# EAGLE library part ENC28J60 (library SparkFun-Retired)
Microchip SPI 10Base ethernet IC Prototype by abe, 2010. Dead?
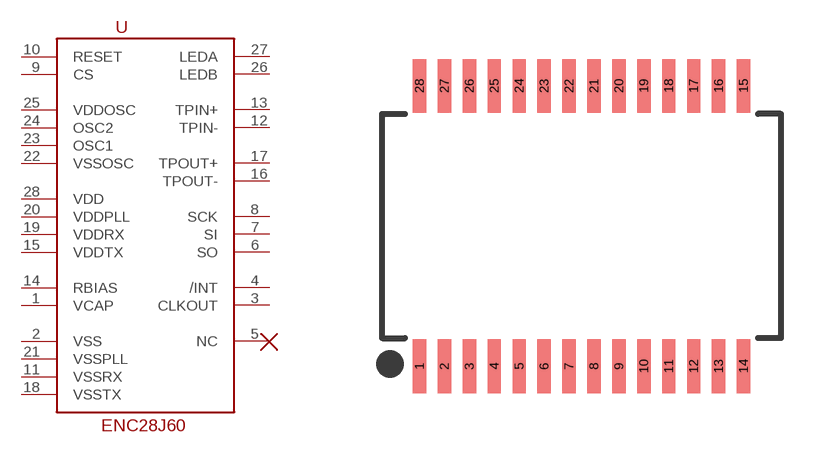
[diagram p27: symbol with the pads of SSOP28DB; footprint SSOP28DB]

Designator prefix U

## ENC28J60 (PROD_ID: IC-09541; VALUE: ENC28J60)  [SSOP28DB]
1  VCAP
2  VSS
3  CLKOUT
4  /INT
5  NC
6  SO
7  SI
8  SCK
9  CS
10  RESET
11  VSSRX
12  TPIN-
13  TPIN+
14  RBIAS
15  VDDTX
16  TPOUT-
17  TPOUT+
18  VSSTX
19  VDDRX
20  VDDPLL
21  VSSPLL
22  VSSOSC
23  OSC1
24  OSC2
25  VDDOSC
26  LEDB
27  LEDA
28  VDD

## Footprint SSOP28DB (pad centres in mm)
Small Shrink Outline Package
smd 0.348 x 1.397: 1 -4.225,-3.656; 2 -3.575,-3.656; 3 -2.925,-3.656; 4 -2.275,-3.656; 5 -1.625,-3.656; 6 -0.975,-3.656; 7 -0.325,-3.656; 8 0.325,-3.656; 9 0.975,-3.656; 10 1.625,-3.656; 11 2.275,-3.656; 12 2.925,-3.656; 13 3.575,-3.656; 14 4.225,-3.656; 15 4.225,3.656; 16 3.575,3.656; 17 2.925,3.656; 18 2.275,3.656; 19 1.625,3.656; 20 0.975,3.656; 21 0.325,3.656; 22 -0.325,3.656; 23 -0.975,3.656; 24 -1.625,3.656; 25 -2.275,3.656; 26 -2.925,3.656; 27 -3.575,3.656; 28 -4.225,3.656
